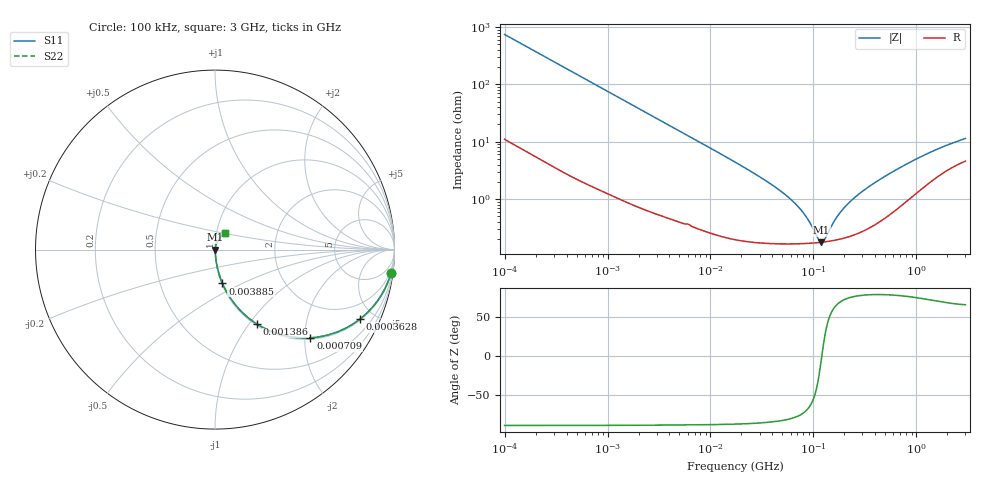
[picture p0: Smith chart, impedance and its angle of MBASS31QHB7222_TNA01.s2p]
! MBASS31QHB7222_TNA01  S-PARAMETER MODEL  ( Standard Model )
! Model Generated by TAIYO YUDEN Corporation (http://www.ty-top.com)
! Version 2.0
! TAIYO YUDEN Control No. 231201
! Copyright(c) 2013 TAIYO YUDEN CO.,LTD. All Rights Reserved.
! Product Description (link to TY-COMPAS)
! https://ds.yuden.co.jp/TYCOMPAS/or/detail?pn=MBASS31QHB7222KTNA01&u=M
! Products Name : Multilayer Ceramic Capacitors
! Characteristics :
!  Capacitance : 2200 [pF] , Rated Voltage : 630 [V] , TCC : X7R
!  Case Size : 3.2 x 1.6 / 0.126 x 0.063 [mm/inch] , Thickness : 1.15 / 0.045 [mm/inch]
!  (Conditions: Temperature = 25 [degC] , DC Bias Voltage = 0 [V])
! External Node Assignments :
!  1  o---| |---o  2
! GND o---------o GND
! Frequency Range : 100kHz  -  3GHz  [ 401 STEP ]
# MHZ S RI R 50
! Freq[MHz].  S11 Real  S11 Imag  S21 Real  S21 Imag  S12 Real  S12 Imag  S22 Real  S22 Imag
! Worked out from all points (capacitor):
!   401 points, 100 kHz to 3 GHz, reference 50 ohm
!   read as one part in series: C = 2.14 nF near 105.3 kHz
!   lowest |Z| = 176 mohm at 119.7 MHz (marker M1)
!   series resonance near 120.7 MHz, so ESL is about 810 pH
!   S11 on the Smith chart (normalised r, x): 100 kHz: 1, -15; 362.8 kHz: 1.06, -4.14; 709 kHz: 1.03, -2.13; 1.386 MHz: 1.02, -1.10; 3.885 MHz: 1.01, -0.40; 3 GHz: 1.09, +0.21
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0.1  0.9803 -0.1316  0.0197 0.1316  0.0197 0.1316  0.9803 -0.1316
0.205778  0.9265 -0.2538  0.0735 0.2538  0.0735 0.2538  0.9265 -0.2538
0.362777  0.8076 -0.387  0.1924 0.387  0.1924 0.387  0.8076 -0.387
0.562235  0.6409 -0.4724  0.3591 0.4724  0.3591 0.4724  0.6409 -0.4724
0.709011  0.5314 -0.4914  0.4686 0.4914  0.4686 0.4914  0.5314 -0.4914
1.385689  0.2353 -0.4156  0.7647 0.4156  0.7647 0.4156  0.2353 -0.4156
2.039661  0.1274 -0.3241  0.8726 0.3241  0.8726 0.3241  0.1274 -0.3241
3.161081  0.0598 -0.2266  0.9402 0.2266  0.9402 0.2266  0.0598 -0.2266
3.884884  0.0416 -0.1884  0.9584 0.1884  0.9584 0.1884  0.0416 -0.1884
17.7727  0.00376 -0.0427  0.9962 0.0427  0.9962 0.0427  0.00376 -0.0427
55.23785  0.00177 -0.0112  0.9982 0.0112  0.9982 0.0112  0.00177 -0.0112
77.22239  0.0017 -0.00596  0.9983 0.00596  0.9983 0.00596  0.0017 -0.00596
97.38194  0.00171 -0.00279  0.9983 0.00279  0.9983 0.00279  0.00171 -0.00279
110.7752  0.00173 -0.00111  0.9983 0.00111  0.9983 0.00111  0.00173 -0.00111
119.6798  0.00175 -0.000112  0.9982 0.000112  0.9982 0.000112  0.00175 -0.000112
129.3002  0.00179 0.000885  0.9982 -0.000885  0.9982 -0.000885  0.00179 0.000885
171.6802  0.00197 0.00463  0.998 -0.00463  0.998 -0.00463  0.00197 0.00463
216.4987  0.00223 0.00793  0.9978 -0.00793  0.9978 -0.00793  0.00223 0.00793
318.6746  0.00306 0.0144  0.9969 -0.0144  0.9969 -0.0144  0.00306 0.0144
547.5153  0.00594 0.0268  0.9941 -0.0268  0.9941 -0.0268  0.00594 0.0268
1315.078  0.0217 0.0581  0.9783 -0.0581  0.9783 -0.0581  0.0217 0.0581
3000  0.0532 0.0946  0.9468 -0.0946  0.9468 -0.0946  0.0532 0.0946
